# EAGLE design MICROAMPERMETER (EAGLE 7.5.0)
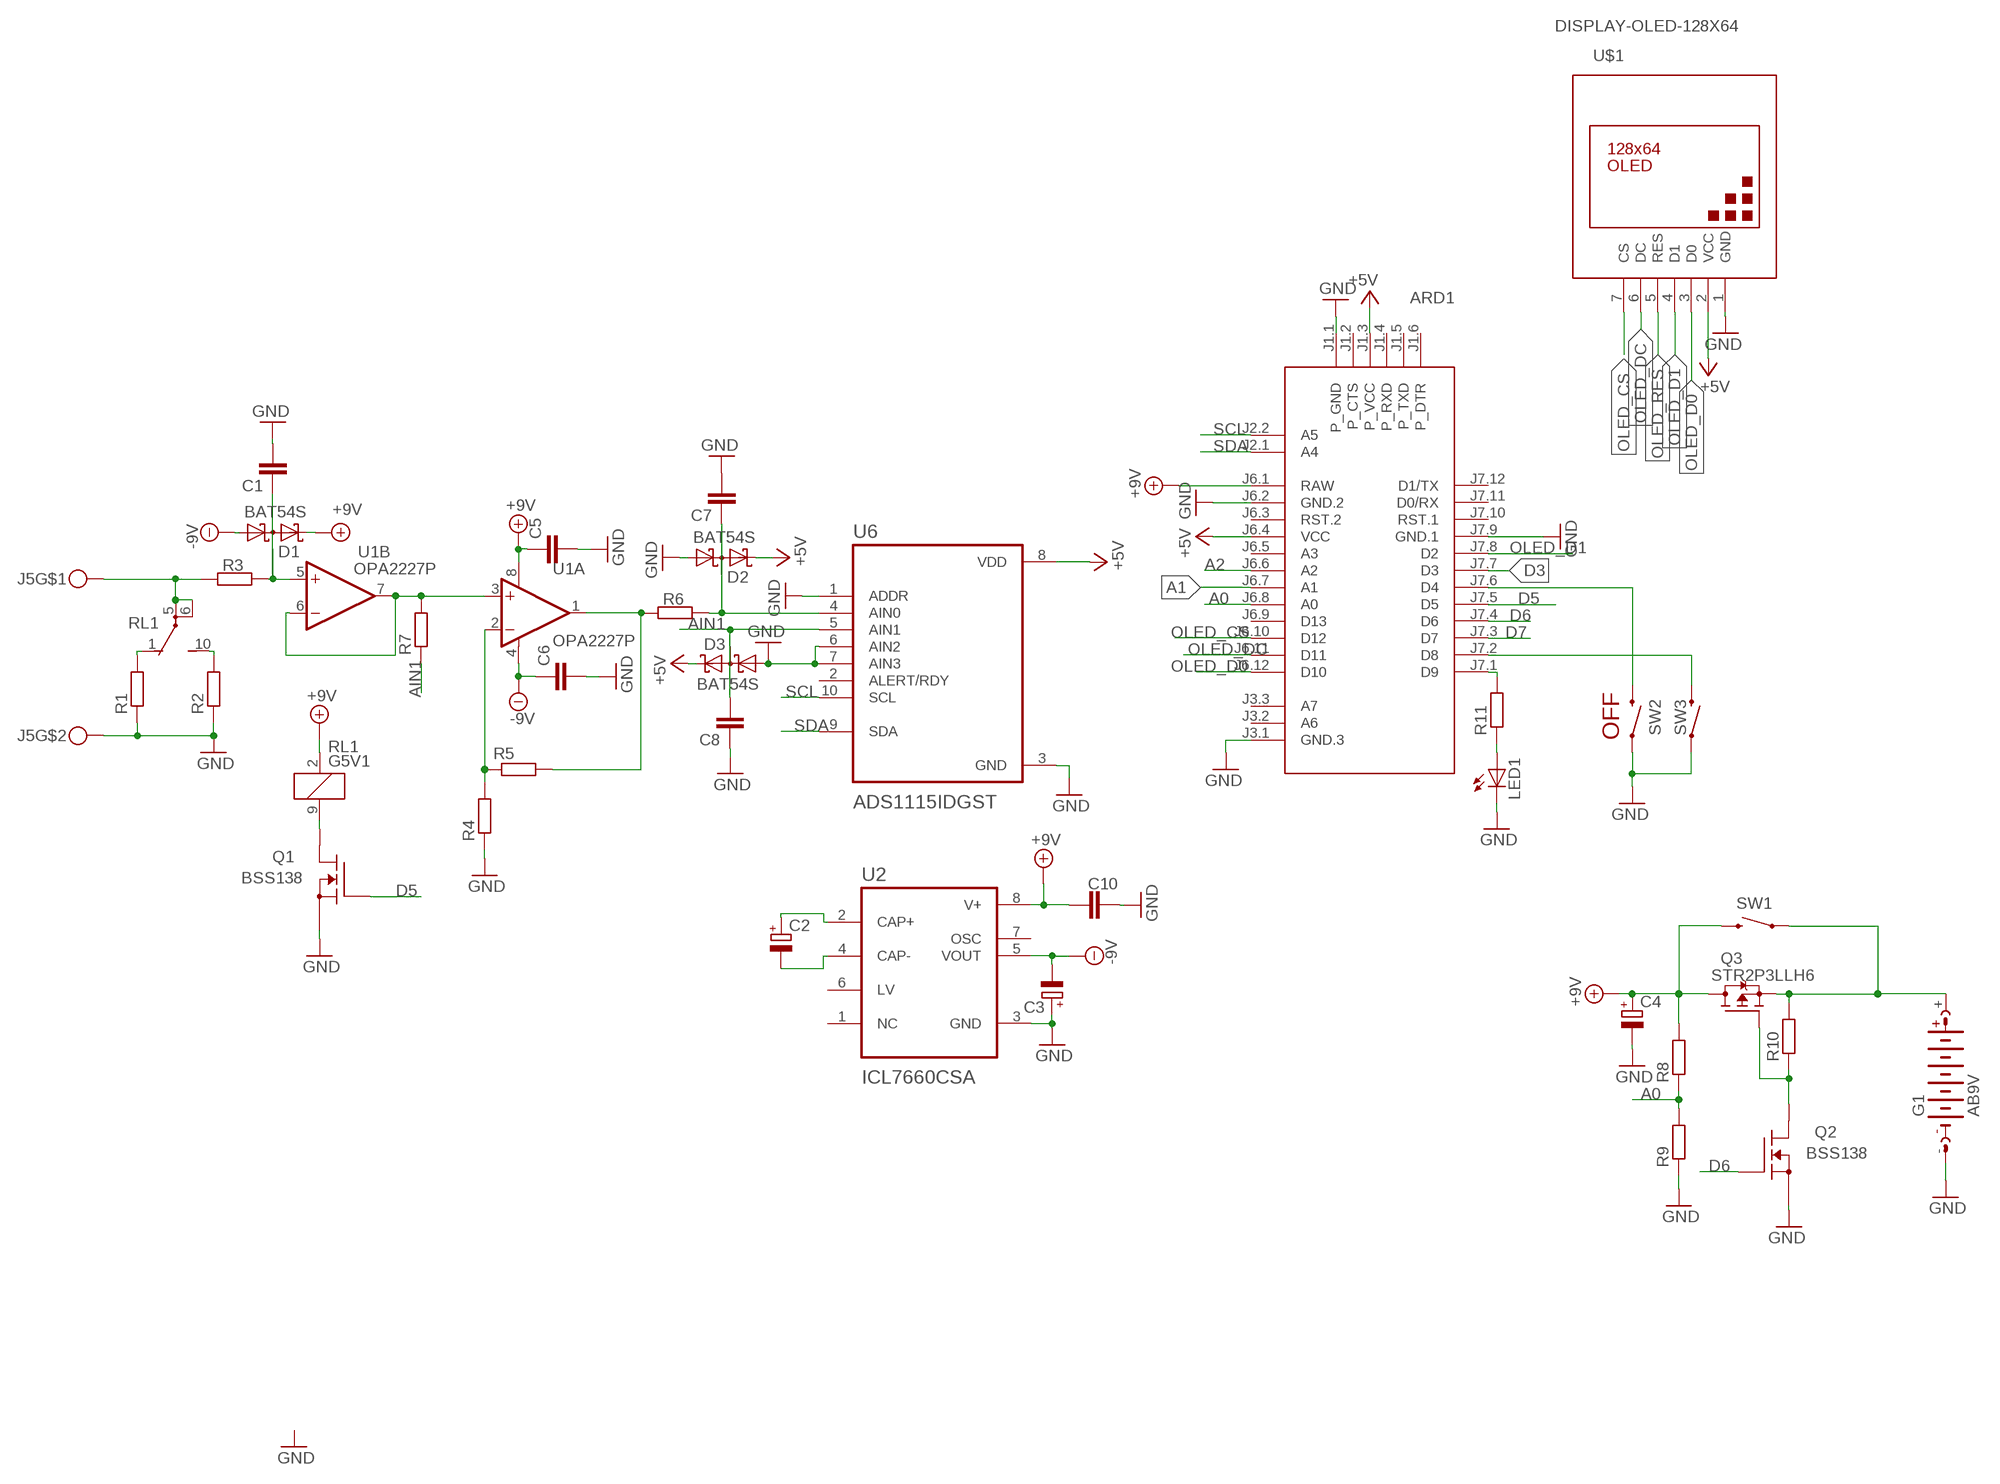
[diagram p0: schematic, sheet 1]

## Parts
ARD1  ARDUINO-PRO-MINI-3.3V  [ARDUINO-PRO-MINI]
C1  C-EUC1206  [C1206]
C2  CPOL-EUSMCC  [SMC_C]
C3  CPOL-EUSMCC  [SMC_C]
C4  CPOL-EUSMCC  [SMC_C]
C5  C-EUC1206  [C1206]
C6  C-EUC1206  [C1206]
C7  C-EUC1206  [C1206]
C8  C-EUC1206  [C1206]
C10  C-EUC1206  [C1206]
D1  BAT54S  [SOT23]
D2  BAT54S  [SOT23]
D3  BAT54S  [SOT23]
G1  AB9V  [AB9V]
J5  MKDSN1,5-2-5,08  [MKDSN1,5-2-5,08]
LED1  LED5MM  [LED5MM]
Q1  BSS138  [SOT23]
Q2  BSS138  [SOT23]
Q3  STR2P3LLH6  [SOT23]
R1  R-EU_0207/10  [0207/10]
R2  R-EU_0207/10  [0207/10]
R3  R-EU_R1206  [R1206]
R4  R-EU_0207/10  [0207/10]
R5  R-EU_0207/10  [0207/10]
R6  R-EU_R1206  [R1206]
R7  R-EU_R1206  [R1206]
R8  R-EU_R1206  [R1206]
R9  R-EU_R1206  [R1206]
R10  R-EU_R1206  [R1206]
R11  R-EU_R1206  [R1206]
RL1  G5V1  [G5V1]
SW1  SWITCH-MOMENTARY-2SMD  [TACTILE-SWITCH-SMD]
SW2  SWITCH-MOMENTARY-2SMD  [TACTILE-SWITCH-SMD]
SW3  SWITCH-MOMENTARY-2SMD  [TACTILE-SWITCH-SMD]
U1  OPA2227P  OPA2234P  [DIL08]
U2  ICL7660CSA  [SOIC127P600X175-8N]
U6  ADS1115IDGST  [SOP50P490X110-10N]
U$1  DISPLAY-OLED-128X64  [DISPLAY-OLED-128X64]

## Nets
+5V: ARD1.J1.3(P_VCC) ARD1.J6.4(VCC) D2.2(C2) D3.2(C2) U6.8(VDD) U$1.2(VCC)
+9V: ARD1.J6.1(RAW) C4.+ C5.1 C10.2 D1.2(C2) Q3.1(D) R8.2 RL1.2 SW1.3 U1.8(A:V+) U2.8(V+)
-9V: C3.- C6.1 D1.1(A1) U1.4(A:V-) U2.5(VOUT)
A0: ARD1.J6.8(A0) R8.1 R9.2
A1: ARD1.J6.7(A1)
A2: ARD1.J6.6(A2)
AIN1: C8.2 D3.3(C1A2) R7.1 U6.5(AIN1)
D3: ARD1.J7.7(D3)
D5: ARD1.J7.5(D5) Q1.3(G)
D6: ARD1.J7.4(D6) Q2.3(G)
D7: ARD1.J7.3(D7)
GND: ARD1.J1.1(P_GND) ARD1.J3.1(GND.3) ARD1.J6.2(GND.2) ARD1.J7.9(GND.1) C1.2 C3.+ C4.- C5.2 C6.2 C7.2 C8.1 C10.1 D2.1(A1) D3.1(A1) G1.- J5.2 LED1.K(C) Q1.1(S) Q2.1(S) R1.1 R2.1 R4.1 R9.1 SW2.1 SW3.1 U2.3(GND) U6.1(ADDR) U6.3(GND) U6.6(AIN2) U6.7(AIN3) U$1.1(GND)
N$1: R4.2 R5.1 U1.2(A:-IN)
N$2: C7.1 D2.3(C1A2) R6.1 U6.4(AIN0)
N$3: R5.2 R6.2 U1.1(A:OUT)
N$4: R7.2 U1.3(A:+IN) U1.6(B:-IN) U1.7(B:OUT)
N$5: C1.1 D1.3(C1A2) R3.1 U1.5(B:+IN)
N$6: J5.1 R3.2 RL1.5(2:P) RL1.6(2:P)
N$7: R1.2 RL1.1(2:O)
N$8: R2.2 RL1.10(2:S)
N$10: Q1.2(D) RL1.9
N$17: ARD1.J7.1(D9) R11.2
N$18: ARD1.J7.6(D4) SW2.3
N$19: Q2.2(D) Q3.2(G) R10.1
N$20: G1.+ Q3.3(S) R10.2 SW1.1
N$21: LED1.A R11.1
N$23: C2.+ U2.2(CAP+)
N$24: C2.- U2.4(CAP-)
N$27: ARD1.J7.2(D8) SW3.3
OLED_CS: ARD1.J6.10(D12) U$1.7(CS)
OLED_D0: ARD1.J6.12(D10) U$1.3(D0)
OLED_D1: ARD1.J7.8(D2) U$1.4(D1)
OLED_DC: ARD1.J6.11(D11) U$1.6(DC)
OLED_RES: U$1.5(RES)
SCL: ARD1.J2.2(A5) U6.10(SCL)
SDA: ARD1.J2.1(A4) U6.9(SDA)
Unconnected: ARD1.J1.2(P_CTS) ARD1.J1.4(P_RXD) ARD1.J1.5(P_TXD) ARD1.J1.6(P_DTR) ARD1.J3.2(A6) ARD1.J3.3(A7) ARD1.J6.3(RST.2) ARD1.J6.5(A3) ARD1.J6.9(D13) ARD1.J7.10(RST.1) ARD1.J7.11(D0/RX) ARD1.J7.12(D1/TX) U2.1(NC) U2.6(LV) U2.7(OSC) U6.2(ALERT/RDY)

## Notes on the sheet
- OFF

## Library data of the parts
ARD1 = diy-modules:ARDUINO-PRO-MINI-*: Arduino Pro Mini and compatible devices More details available here: https://www.arduino.cc/en/Main/ArduinoBoardProMini Click here to find device on ebay.com
C1 C5-C8 C10 = rcl:C-EU: CAPACITOR, European symbol
C2-C4 = rcl:CPOL-EU: POLARIZED CAPACITOR, European symbol
D1-D3 = diode:BAT54S: Schottky Diodes Pin connection corrected 2011-05-04 Source: Fairchild .. BAT54.pdf
G1 = battery:AB9V: 9-V BATTERY CLIP
J5 = con-phoenix-508:MKDSN1,5-2-5,08
LED1 = led:LED: LED
Q1 Q2 = transistor-fet:BSS138
Q3 = transistor-fet:STR2P3LLH6
R1-R11 = rcl:R-EU_: RESISTOR, European symbol
RL1 = relay:G5V1: RELAY 1 x switch, 0.5 A/125 V AC, 1 A/24 V DC , Omron; MPN: G5V-1-DC24; OC_FARNELL: 9949593; OC_NEWARK: 36M6377
SW1-SW3 = SparkFun-Electromechanical:SWITCH-MOMENTARY-2: Various NO switches- pushbuttons, reed, etc; PROD_ID: SWCH-08247
U1 = burr-brown:OPA2234: Operational Amplifier; OC_FARNELL: unknown; OC_NEWARK: unknown
U2 = ICL7660CSA:ICL7660CSA: Check availability; AVAILABILITY: In Stock; CHECK_PRICES: https://www.snapeda.com/parts/ICL7660CSA/Analog+Devices/view-part/?ref=eda; DESCRIPTION: Charge Pump Switching Regulator IC Positive or Negative Fixed -Vin, nVin, Vin/2 1 Output 20mA 8-SOIC (0.154, 3.90mm Width); MF: Analog Devices; MP: ICL7660CSA; PACKAGE: SOIC-8 Maxim; PRICE: None; SNAPEDA_LINK: https://www.snapeda.com/parts/ICL7660CSA/Analog+Devices/view-part/?ref=snap
U6 = ADS1115IDGST:ADS1115IDGST: Check availability; AVAILABILITY: In Stock; CHECK_PRICES: https://www.snapeda.com/parts/ADS1115IDGST/Texas+Instruments/view-part/?ref=eda; DESCRIPTION: 16-bit, 860-SPS, 4-channel, delta-sigma ADC with PGA, oscillator, VREF, comparator and I2C; MF: Texas Instruments; MP: ADS1115IDGST; PACKAGE: VSSOP-10 Texas Instruments; PRICE: None; SNAPEDA_LINK: https://www.snapeda.com/parts/ADS1115IDGST/Texas+Instruments/view-part/?ref=snap
U$1 = diy-modules:DISPLAY-OLED-128X64: 128x64 Dot Matrix OLED Module based on SSD1306 chip Variant with SPI interface More details available here: http://www.instructables.com/id/How-to-use-OLED-display-arduino-module/ SSD1306 datasheet: https://cdn-shop.adafruit.com/datasheets/SSD1306.pdf Click here to find device on ebay.com Note: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

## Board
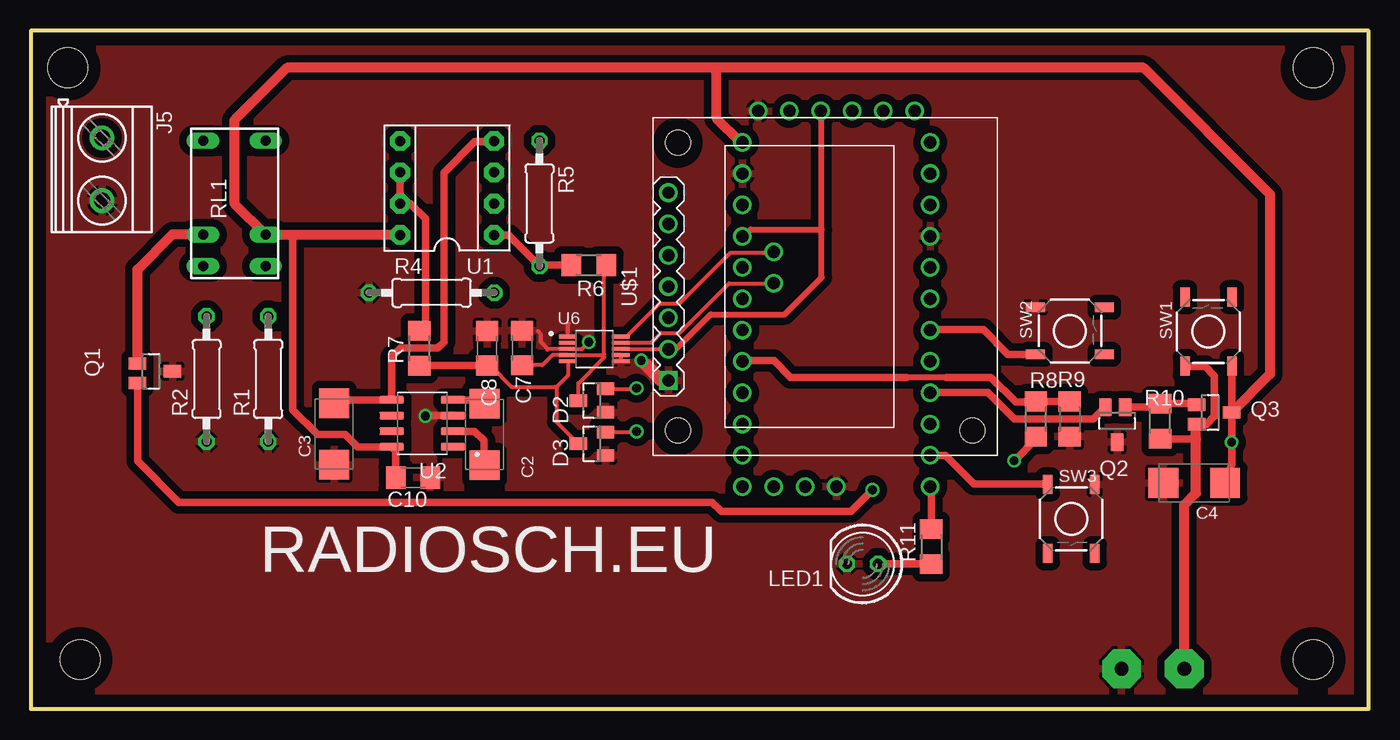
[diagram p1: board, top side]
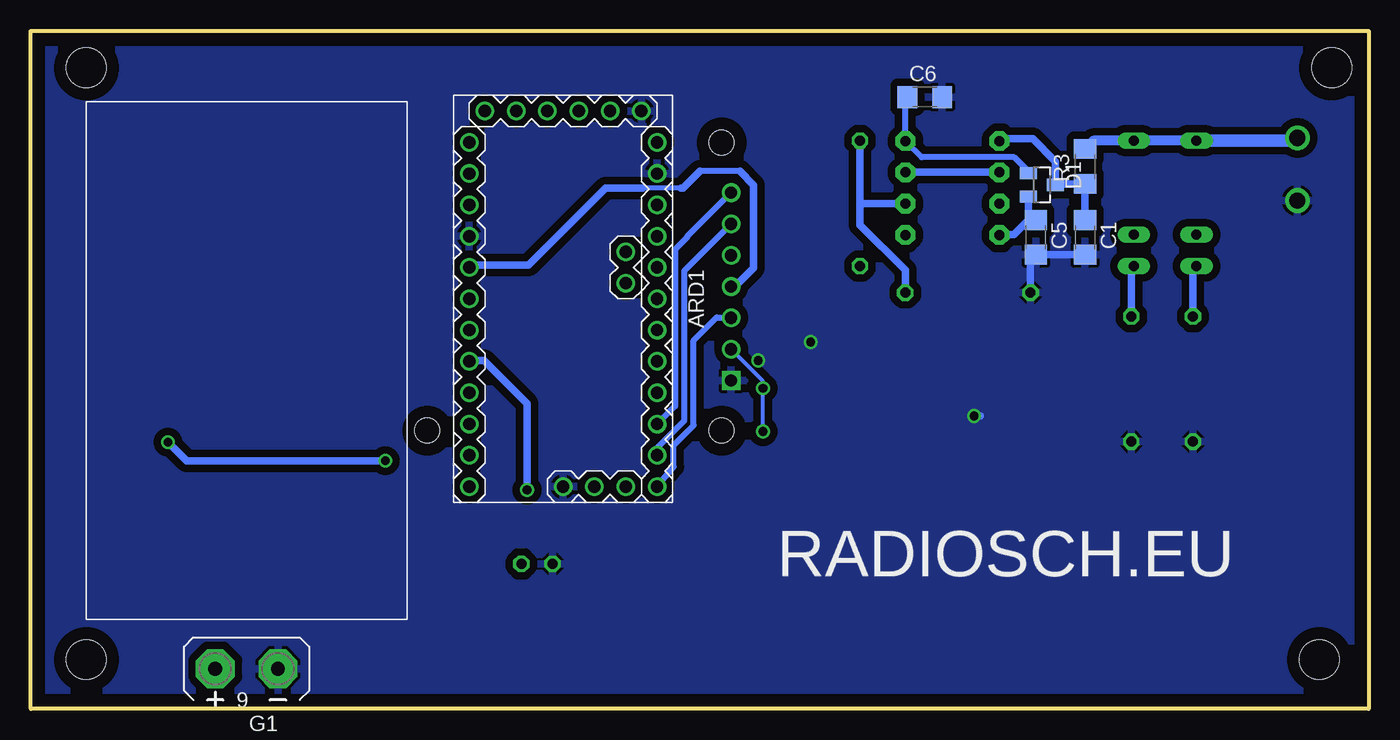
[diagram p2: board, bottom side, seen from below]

Size 108.5 x 55 mm. Coordinates in mm from the lower left corner, seen from the top.
Outline: 0,0 108.5,0 108.5,55 0,55 0,0
Copper layers (1*16): Top 0.035mm / dielectric 1.5mm / Bottom 0.035mm
Design rules "default *": minimum track width 10mil, minimum drill 24mil, track to track 6mil, track to pad 6mil, pad to pad 6mil, via to via 8mil, smd to smd 8mil, copper to edge 40mil, drill to drill 8mil, minimum pad ring 10mil, minimum via ring 8mil, stop-mask expansion 4mil, vias tented up to drill 0mil, thermal gap 10mil
Holes 3.2 mm at 3,52 4,4 104,4 104,52

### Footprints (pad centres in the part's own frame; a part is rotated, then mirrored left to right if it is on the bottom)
ARDUINO-PRO-MINI = drill 1: J1.1 -15.24,6.35; J1.2 -15.24,3.81; J1.3 -15.24,1.27; J1.4 -15.24,-1.27; J1.5 -15.24,-3.81; J1.6 -15.24,-6.35; J2.1 -1.27,5.08; J2.2 -3.81,5.08; J3.1 15.24,0; J3.2 15.24,2.54; J3.3 15.24,5.08; J6.1 -12.7,7.62; J6.2 -10.16,7.62; J6.3 -7.62,7.62; J6.4 -5.08,7.62; J6.5 -2.54,7.62; J6.6 0,7.62; J6.7 2.54,7.62; J6.8 5.08,7.62; J6.9 7.62,7.62; J6.10 10.16,7.62; J6.11 12.7,7.62; J6.12 15.24,7.62; J7.1 15.24,-7.62; J7.2 12.7,-7.62; J7.3 10.16,-7.62; J7.4 7.62,-7.62; J7.5 5.08,-7.62; J7.6 2.54,-7.62; J7.7 0,-7.62; J7.8 -2.54,-7.62; J7.9 -5.08,-7.62; J7.10 -7.62,-7.62; J7.11 -10.16,-7.62; J7.12 -12.7,-7.62
C1206 = smd 1.6 x 1.8: 1 -1.4,0; 2 1.4,0
SMC_C = smd 2.4 x 2.4: + -2.5,0; - 2.5,0
SOT23 = smd 1 x 1.4: 1 -0.95,-1.1; 2 0.95,-1.1; 3 0,1.1
AB9V = drill 1.118 pad 3.15 octagon: + 0,2.54; - 0,-2.54
MKDSN1,5-2-5,08 = drill 1.3 pad 2: 1 -2.561,0.025; 2 2.519,0.025
LED5MM = drill 0.813 octagon: A -1.27,0; K 1.27,0
SOT23' = smd 1 x 1.4: 1 0,1.735; 2 -0.632,-1.1; 3 0.95,-1.1
0207/10 = drill 0.813 octagon: 1 -5.08,0; 2 5.08,0
R1206 = smd 1.6 x 1.803: 1 -1.422,0; 2 1.422,0
G5V1 = drill 0.813 long: 1 -5.08,-2.54; 2 -2.54,-2.54; 5 5.08,-2.54; 6 5.08,2.54; 9 -2.54,2.54; 10 -5.08,2.54
TACTILE-SWITCH-SMD = smd 1.524 x 0.762: 1 -2.794,1.905; 2 2.794,1.905; 3 -2.794,-1.905; 4 2.794,-1.905
DIL08 = drill 0.813 pad 1.6 octagon: 1 -3.81,-3.81; 2 -1.27,-3.81; 3 1.27,-3.81; 4 3.81,-3.81; 5 3.81,3.81; 6 1.27,3.81; 7 -1.27,3.81; 8 -3.81,3.81
SOIC127P600X175-8N = smd 1.97 x 0.59: 1 -2.475,1.905; 2 -2.475,0.635; 3 -2.475,-0.635; 4 -2.475,-1.905; 5 2.475,-1.905; 6 2.475,-0.635; 7 2.475,0.635; 8 2.475,1.905
SOP50P490X110-10N = smd 1.47 x 0.28: 1 -2.15,1; 2 -2.15,0.5; 3 -2.15,0; 4 -2.15,-0.5; 5 -2.15,-1; 6 2.15,-1; 7 2.15,-0.5; 8 2.15,0; 9 2.15,0.5; 10 2.15,1
DISPLAY-OLED-128X64 = drill 1 square: 1 -7.62,12.7 | drill 1: 2 -5.08,12.7; 3 -2.54,12.7; 4 0,12.7; 5 2.54,12.7; 6 5.08,12.7; 7 7.62,12.7 | hole 2: -11.684,11.938; 11.684,11.938; -11.684,-11.938

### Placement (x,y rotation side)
ARD1  65.33,33.26 270 bottom
C1  23,38.25 270 bottom
C2  36.8,22.25 90 top
C3  24.6,22.3 90 top
C4  94.35,18.32 180 top
C5  27,38.25 270 bottom
C6  36,49.62 0 bottom
C7  39.85,29.27 90 top
C8  37,29.25 270 top
C10  31,18.75 180 top
D1  26.5,42.5 270 bottom
D2  45.5,25 90 top
D3  45.5,21.5 90 top
G1  91,3.25 90 bottom
J5  5.75,43.75 270 top
LED1  67.45,11.75 180 top
Q1  BSS138  [SOT23']  9.75,27.38 270 top
Q2  BSS138  [SOT23']  88.1,23.37 180 top
Q3  STR2P3LLH6  [SOT23']  95.64,24.04 270 top
R1  19.25,26.75 90 top
R2  14.25,26.75 90 top
R3  23,44 90 bottom
R4  32.5,33.75 0 top
R5  41.25,41 270 top
R6  45.25,36 180 top
R7  31.5,29.25 90 top
R8  81.5,23.5 270 top
R9  84.25,23.5 90 top
R10  91.58,23.33 270 top
R11  73.03,13.15 90 top
RL1  16.5,41 90 top
SW1  95.5,30.6 90 top
SW2  84.28,30.65 0 top
SW3  84.38,15.4 270 top
U1  33.75,42.25 90 top
U2  31.75,23.15 180 top
U6  45.7,29.2 0 top
U$1  64.41,34.25 90 top

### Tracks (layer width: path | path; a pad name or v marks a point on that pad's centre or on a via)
+5V  (via drill 0.7)
  Top 0.305: U6.8 51.68,29.2 U$1.2 | D2.2 49.08,25.95 v49.12,26 | D3.2 49.08,22.45 v49.12,22.5
  Top 0.5: 51.68,29.2 52.33,29.2 55.12,32 61.12,32 64.12,35 64.12,38.88 | 64.12,38.88 64.12,48.44 ARD1.J1.3 | ARD1.J6.4 57.84,38.34 58.38,38.88 64.12,38.88
  Bottom 0.305: U$1.2 49.12,26.59 v49.12,26 v49.12,22.5
+9V  (via drill 0.7)
  Top 0.61: SW1.3 97.38,27.78 Q3.1 v97.38,21.62 97.38,19.86 C4.+ | R8.2 81.5,21.88 v79.75,20.12 | C10.2 29.6,20.92 U2.8 26.75,21.25 26.5,21.25 25.5,22.25 23.25,22.25 21.25,24.25 21.25,38.21 21.5,38.46
  Top 0.813: ARD1.J6.1 57.54,45.96 55.62,47.88 55.62,51.75 55.38,52 | Q3.1 100.5,27.16 100.5,41.75 90.25,52 55.38,52 | 55.38,52 20.75,52 16.5,47.75 16.5,41 RL1.2 21.5,38.46 29.92,38.46 U1.8
  Bottom 0.61: v79.75,20.12 95.88,20.12 v97.38,21.62 | D1.2 27.6,40.25 C5.1 27.15,39.5 27.75,39.5 28.79,38.46 29.92,38.46 U1.8
-9V
  Top 0.61: C3.- 24.86,25.05 U2.5 29.27,28.52 30,29.25 33,29.25 33.5,29.75 33.5,43.5 36,46 37.5,46 U1.4
  Bottom 0.5: D1.1 27.6,43.6 28.75,44.75 36.25,44.75 U1.4 37.56,49.47 C6.1
A0
  Top 0.5: 74.25,26.88 71,26.88
  Top 0.61: R9.2 R8.1 81.5,24.88 79.88,24.88 77.88,26.88 74.25,26.88 | 71,26.88 61.62,26.88 60.25,28.25 57.78,28.25 ARD1.J6.8
AIN1
  Top 0.305: U6.5 43.55,27.05 42.62,26.12 42.62,26 | 42.62,26 42.62,23.27 D3.3 | C8.2 37.27,27.85 39,26.12 42.5,26.12 42.62,26
  Top 0.61: R7.1 36.98,27.83 C8.2
D5  (via drill 0.7)
  Top 0.61: Q1.3 8.65,20.1 12,16.75 55.25,16.75 56,16 66.5,16 v68.25,17.75
  Bottom 0.61: v68.25,17.75 68.25,24.75 71.75,28.25 72.88,28.25 ARD1.J7.5
D6
  Top 0.61: Q2.3 86.18,23.5 79.75,23.5 77.61,25.64 ARD1.J7.4
GND  (via drill 0.7)
  Top 0.305: U6.6 U6.7 | U6.1 43.55,31.18 43.62,31.25 | U6.3 41.95,29.2 41.88,29.12 | U6.3 41.92,29.2 41.38,29.75 41.38,30.38 41.12,30.62 | U6.3 44.7,29.2 v45.25,29.75
  Top 0.61: U2.3 32.03,23.79 v32,23.75
  Top 1.016: U$1.1 51.12,26.63 49.88,27.88
  Bottom 0.61: C1.2 C5.2 27.42,36.43 R4.1 | v32,23.75 31.5,23.75
  other vias: 49.5,28.25
  pour Top (isolate 0.61): 1,54 108,54 108,1 1,1
  pour Bottom (isolate 0.61): 1,54 108,54 108,1 1,1
N$1
  Bottom 0.61: R4.2 37.58,35.58 41.25,39.25 41.25,41 | 41.25,41 R5.1 | U1.2 41.23,40.98 41.25,41
N$2
  Top 0.305: D2.3 44.4,26.4 46.5,28.5 46.5,28.75 | C7.1 41.5,27.88 42.33,28.7 U6.4 46.45,28.7 46.5,28.75 | 46.5,28.75 46.5,35.83 R6.1
N$3
  Top 0.61: R6.2 41.33,36 R5.2 38.73,38.44 U1.1
N$4
  Top 0.61: U1.6 U1.7 29.96,41 30.75,41 32,39.75 32,31 31.67,30.67 R7.2
  Bottom 0.61: U1.6 U1.3
N$5
  Bottom 0.61: C1.1 R3.1 25.32,42.58 D1.3 25.4,44.4 27.25,46.25 29.75,46.25 U1.5
N$6
  Bottom 0.813: RL1.6 RL1.5 22.34,46.08 R3.2
  Bottom 1.016: RL1.6 6.01,46.08 J5.1
N$7
  Bottom 0.61: R1.2 19.25,35.71 RL1.1
N$8
  Bottom 0.61: R2.2 14.25,35.63 RL1.10
N$10
  Top 0.813: Q1.2 8.65,35.65 11.5,38.5 13.92,38.5 RL1.9
N$17
  Top 0.61: R11.2 73.03,17.95 ARD1.J7.1
N$18
  Top 0.61: SW2.3 79.25,28.75 77.25,30.75 72.98,30.75 ARD1.J7.6
N$19
  Top 0.61: 94.41,24.53 Q3.2 94.46,24.75 R10.1 91.3,24.47 Q2.2
N$20
  Top 0.61: Q3.3 95.33,23.09 96,23.75 96,27 95.25,27.75 93.65,27.75 SW1.1 | R10.2 94.47,21.91 94.5,21.88
  Top 0.813: G1.+ 93.54,16.54 94.5,17.5 94.5,21.88 94.5,23.04 Q3.3
N$21
  Top 0.61: LED1.A 73,11.75 R11.1
N$23
  Top 0.61: U2.2 35.98,22.52 36.75,21.75 36.75,19.8 C2.+
N$24
  Top 0.61: U2.4 36.49,25.05 C2.-
N$27
  Top 0.61: ARD1.J7.2 74.19,20.56 76.5,18.25 82.41,18.25 SW3.3
OLED_CS
  Bottom 0.5: U$1.7 55.25,38.33 55.25,38.25 56.25,37.25 56.25,24.56 ARD1.J6.10
OLED_D0
  Bottom 0.5: ARD1.J6.12 56.38,19.62 56.38,21.38 54.75,23 54.75,29.88 52.88,31.75 51.75,31.75 U$1.3
OLED_D1
  Bottom 0.406: 55.75,42.25 58.88,42.25
  Bottom 0.5: 51,43.62 54.25,43.62
  Bottom 0.61: U$1.4 51.38,34.25 49.88,35.75 49.88,42.5 51,43.62 | 54.25,43.62 55.62,42.25 55.75,42.25 | 58.88,42.25 61.88,42.25 68.12,36 72.75,36 ARD1.J7.8
OLED_DC
  Bottom 0.5: ARD1.J6.11 57.71,21.16 55.5,23.38 55.5,35.54 U$1.6
SCL
  Top 0.305: U6.10 48.33,30.2 51,32.88 52.62,32.88 56.75,37 60.18,37 ARD1.J2.2
SDA
  Top 0.305: U6.9 50.33,29.7 51.12,30.5 52.62,30.5 56.62,34.5 60.22,34.5 ARD1.J2.1

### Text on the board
tPlace: RADIOSCH.EU
bPlace: RADIOSCH.EU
